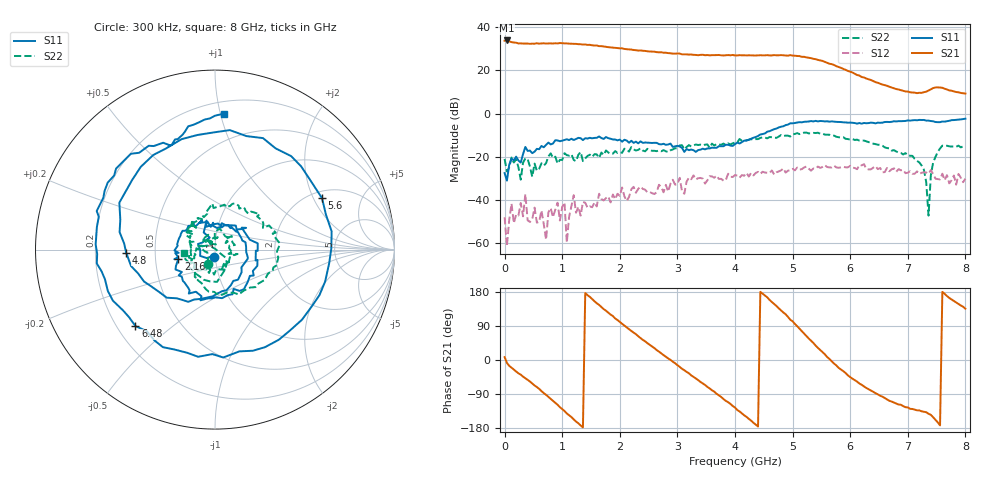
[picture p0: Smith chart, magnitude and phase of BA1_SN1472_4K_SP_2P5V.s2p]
! VC=2.5V IC=18.73mA
# HZ S DB R 50.00
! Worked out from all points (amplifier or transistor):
!   201 points, 300 kHz to 8 GHz, reference 50 ohm
!   highest |S21| = 33.9 dB at 40.3 MHz (marker M1)
!   |S21| within 3 dB of that: start of sweep to 1.772 GHz
!   unconditionally stable (mu >= 1): start of sweep to 3.025 GHz; 3.047 GHz to 3.186 GHz; 6.264 GHz to end of sweep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
!   at 1.32 GHz: K = 2.70, MAG = 32.6 dB, |S12| = -47.4 dB
!   at 4 GHz: K = 0.93, MSG = 27.8 dB, |S12| = -28.6 dB
!   at 8 GHz: K = 2.23, MAG = 13.5 dB, |S12| = -30.3 dB
!   S11 on the Smith chart (normalised r, x): 300 kHz: 0.99, -0.08; 2.16 GHz: 0.66, -0.07; 4.8 GHz: 0.34, -0.02; 5.6 GHz: 2.30, +2.34; 6.48 GHz: 0.27, -0.38; 8 GHz: 0.29, +1.02
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300000  -27.65 -96.1  33.82 7.6  -48.13 -24.3  -21.09 -114.9
4.02985e7  -31.13 -91.1  33.93 -7.5  -61.56 -92.7  -26.87 -160.7
3.20288e8  -18.86 123.5  32.49 -44.0  -47.73 -122.6  -22.85 129.4
6.802745e8  -15.66 43.0  32.61 -87.4  -51.36 10.7  -24.22 105.8
8.80267e8  -12.38 8.3  32.63 -112.8  -44.59 129.8  -20.02 40.5
1.08026e9  -11.95 -21.0  32.57 -141.1  -59.87 100.5  -19.32 30.6
1.360249e9  -12.31 -64.6  32.02 -177.8  -41.04 -5.1  -22.07 -17.0
1.720236e9  -11.77 -114.3  31.12 134.3  -40.32 7.0  -19.21 -85.6
2.160219e9  -13.54 -166.1  29.79 81.6  -38.76 4.7  -17.68 -143.7
2.6802e9  -14.20 147.5  28.44 22.0  -33.07 -66.0  -17.15 175.8
3.040186e9  -15.29 120.5  27.84 -18.1  -29.84 -89.4  -14.79 153.3
3.440171e9  -16.31 61.1  27.29 -61.8  -30.20 -134.6  -14.81 131.2
4.00015e9  -14.21 -40.4  26.96 -125.5  -28.58 -178.1  -13.45 101.5
4.440134e9  -9.71 -117.1  27.07 179.8  -28.00 136.8  -11.30 69.3
4.80012e9  -6.10 -178.1  27.13 130.9  -26.37 97.4  -9.95 38.4
5.120108e9  -4.02 123.1  26.69 82.4  -26.00 69.4  -9.54 15.6
5.360099e9  -3.66 74.5  25.40 45.0  -25.50 56.1  -8.98 -7.4
5.60009e9  -3.59 25.6  23.60 7.9  -24.85 24.2  -9.80 -28.8
5.960076e9  -4.23 -47.2  19.78 -40.7  -24.99 -11.9  -11.85 -70.1
6.480057e9  -4.22 -136.1  14.29 -90.7  -25.81 -68.2  -14.50 -118.8
6.68005e9  -3.94 -164.8  12.43 -107.7  -26.80 -77.2  -16.13 -136.7
8e9  -2.39 86.3  9.27 135.5  -30.25 166.6  -15.27 -173.1
